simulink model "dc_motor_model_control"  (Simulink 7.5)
settings: Solver=FixedStepDiscrete  StartTime=0.0  StopTime=60  FixedStep=0.001  RelTol=1e-3
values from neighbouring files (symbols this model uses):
  bits = 32    [hexcalc.m]
undefined symbols (not defined in the file or in its folder): bin2dec, Buffer, characters, contain, DiscIntNeverNeededParam, full, is, PWM, Receive, When
libraries: dsPICdrivers x9, simulink x2

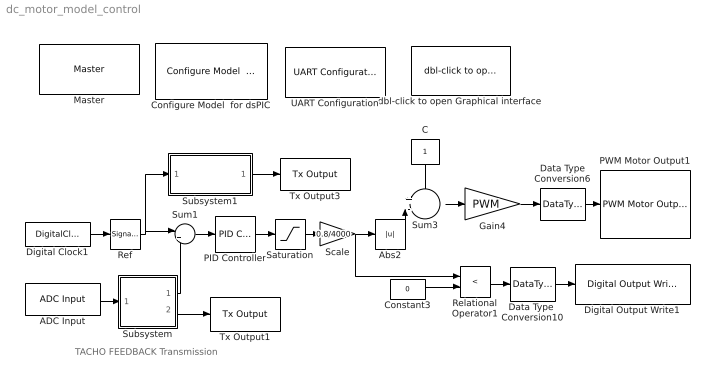
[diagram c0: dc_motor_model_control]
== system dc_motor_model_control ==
  note: TACHO FEEDBACK Transmission
  ADC Input : dsPICdrivers/Peripheral I//O/ADC Input  Tag=dsPIC_ADC  Priority=5  ADC_TYPE=10 bits  ADC_MODE=Continuous sampling & get last channel value  NbrSampleStep=1  VoltRefpopup="AVdd  -  AVss"  OutFormatBitspopup=0000 00dd dddd dddd : Integer  InterruptPriority=6  ANCHANNELS=[3]  MaxName=ANmax = 1023  Rin=1e2  ADCS=1  SAMC=1  Temperature=25  DMAChannel=0  SampleTime=0.001  Status="OK  |  Tsmp=1.600e-007 |  T/Channel=2.080e-006 |  Tall=2.080e-006"  SSRC=auto convert
  Abs2 : Abs  OutDataType=fixdt(1, 16)  OutScaling=2^0
  C : Constant  OutDataType=fixdt(1, 16)  OutScaling=2^0
  Configure Model  for dsPIC : dsPICdrivers/Simulink Configuration/Configure Model  for dsPIC
  Constant3 : Constant  Value=0  OutDataType=fixdt(1, 16)  OutScaling=2^0
  Data Type  Conversion10 : DataTypeConversion  OutDataTypeMode=boolean  OutDataType=fixdt(1, 16)  OutScaling=2^0  OutDataTypeStr=boolean
  Data Type Conversion6 : DataTypeConversion  OutDataTypeMode=uint16  OutDataType=fixdt(1, 16)  OutScaling=2^0  OutDataTypeStr=uint16  SampleTime=0.001
  Digital Clock1 : DigitalClock  SampleTime=0.001
  Digital Output Write1 : dsPICdrivers/Digital I//O/Digital Output Write  Tag=dsPIC_Digital_Output  Priority=5  PORT=D  Pin=[1]  Simultaneous=off  OrderingInOutPopup=None
  Gain4 : Gain  Gain=PWM  ParameterDataType=fixdt(1, 16)  ParameterScaling=2^0  OutDataType=fixdt(1, 16)  OutScaling=2^0  SampleTime=0.001
  Master : dsPICdrivers/Master  Tag=dsPIC_MASTER  Priority=1  TimeStepType=Timer1  picType=30f4012  fcy=6.25e6  Quartz_33f=5e6  PLLActive_33f=off  fcyDesired_33f=0  tmr1="[1  6249  0]"  tmr1Info="Time Step : 0.001  ;   Error : 0%  PR1=6249"  tmr2345="[0  0  0  0]"  tmr2345cfg=[-1 -1 -1 -1]  IOautoConf=on  typePort="[ 0   0   0   0   0   0   0   0   0   0   0   0   0   0   0   0   0   0   0   8   0   0   0   0   0   0   0   0   0   0   0   0   0   0   0   0   0   0   0   0   0   0   0   0   0   0   0   0   0  10   0   0   0   0   0   0   0   0   0   0   0   0   0   0   0   0   0   0   0   0   0   0   0   0   0   0   0   0   0   0   0   0   4   5   0   0   0   0   0   0   0   0   0   0   0   0   0   0   0   0 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"  TRIS="[ 65535  65535  65535  65533  65535  65535  65535 ]"  ADPCFG=0  MasterBusyPort=None  MasterOverloadPort=None  FOSC=HS  ClockSwitchMonitor=Both disabled  TempProtection_33f=TEMP_ON  FPBOR=PBOR_OFF  PWRT=PWRT_OFF  MCLR=MCLR_DIS  ICD=ICS_NONE  JTAGEN=JTAGEN_OFF  PowerSave=off  OverrideFcy=off  NewFcy=1e6  PR2345="[65535  65535  65535  65535]"
  PID Controller : simulink/Continuous/PID Controller  DialogController=pidpack.PIDConfig.pidDDGCreate  DialogControllerArgs=DataTag0  SystemSampleTime=-1  Controller=PID  TimeDomain=Discrete-time  SampleTime=0.001  IntegratorMethod=Forward Euler  FilterMethod=Forward Euler  Form=Parallel  P=2.70860587935341  I=38.2988282363773  D=0.0377965070622529  N=150.289906097433  InitialConditionSource=internal  InitialConditionForIntegrator=0  InitialConditionForFilter=0  ExternalReset=none  LimitOutput=off  UpperSaturationLimit=inf  LowerSaturationLimit=-inf  LinearizeAsGain=off  AntiWindupMode=none  Kb=1  TrackingMode=off  Kt=1  PParamMin=[]  PParamMax=[]  IParamMin=[]  IParamMax=[]  DParamMin=[]  DParamMax=[]  NParamMin=[]  NParamMax=[]  KbParamMin=[]  KbParamMax=[]  KtParamMin=[]  KtParamMax=[]  POutMin=[]  POutMax=[]  IOutMin=[]  IOutMax=[]  DOutMin=[]  DOutMax=[]  NOutMin=[]  NOutMax=[]  KbOutMin=[]  KbOutMax=[]  KtOutMin=[]  KtOutMax=[]  IntegratorOutMin=[]  IntegratorOutMax=[]  FilterOutMin=[]  FilterOutMax=[]  SumOutMin=[]  SumOutMax=[]  SumI1OutMin=[]  SumI1OutMax=[]  SumI2OutMin=[]  SumI2OutMax=[]  SumI3OutMin=[]  SumI3OutMax=[]  SumDOutMin=[]  SumDOutMax=[]  SaturationOutMin=[]  SaturationOutMax=[]  IntegratorContinuousStateAttributes=''  IntegratorStateMustResolveToSignalObject=off  IntegratorRTWStateStorageClass=Auto  FilterContinuousStateAttributes=''  FilterStateMustResolveToSignalObject=off  FilterRTWStateStorageClass=Auto
  PWM Motor Output1 : dsPICdrivers/Peripheral I//O/PWM Motor Output  Tag=dsPIC_PWM_Motor  Priority=5  PWMref=1  PWM12=1  InputEnableChk=off  InputPeriodeChk=off  Channel=[1]  TPeriode=10e-3  PrescalerValue=4  PeriodeInteger=15625  MaxName='PWM'  Centered=off  HChannelON=off  Info="Nbr Bits : 14.9316  ||  PWM = 31250  ||  Prescaler = 4"  Delay=0  IntPriority=5  nbrPwmChannelPIC=3  Status=OK  DeadTimePrescaleA=0  DeadTimePrescaleB=0  DeadTimeInfo=Dead Time A = 0  DTPWM1a=Prescaler A  DTPWM1i=Prescaler A  DTPWM2a=Prescaler A  DTPWM2i=Prescaler A  DTPWM3a=Prescaler A  DTPWM3i=Prescaler A  DTPWM4a=Prescaler A  DTPWM4i=Prescaler A  DTCON1=0  DTCON2=0
  Ref : SignalGenerator  WaveForm=square  TimeSource=Use external signal  Amplitude=2700  Frequency=1/10
  Relational Operator1 : RelationalOperator  Operator=<  LogicOutDataTypeMode=boolean  LogicDataType=fixdt(0, 8)  OutDataTypeStr=boolean
  Saturation : Saturate  UpperLimit=4000  LowerLimit=-4000  OutDataType=fixdt(1, 16)  OutScaling=2^0
  Scale : Gain  Gain=0.8/4000  ParameterDataType=fixdt(1, 16)  ParameterScaling=2^0  OutDataType=fixdt(1, 16)  OutScaling=2^0
  Subsystem : Subsystem
  Subsystem1 : Subsystem
  Sum1 : Sum  Inputs=|+-  OutDataType=fixdt(1, 16)  OutScaling=2^0
  Sum3 : Sum  Inputs=+-  OutDataType=fixdt(1, 16)  OutScaling=2^0
  Tx Output1 : dsPICdrivers/Serial PORT/Tx Output  Tag=dsPIC_TX  Priority=5  UART=1  OrderingInOutPopup=None
  Tx Output3 : dsPICdrivers/Serial PORT/Tx Output  Tag=dsPIC_TX  Priority=5  UART=1  OrderingInOutPopup=None
  UART Configuration : dsPICdrivers/Serial PORT/UART Configuration  Tag=dsPIC_config_UART  Priority=2  UART=1  proposed_BAUD=57600  ALT_TX_RX=off  InterruptTxWhen=When Transmit Buffer is empty  TXInterruptPri=1  TxBufferSize=32  TXEN=on  InterruptRxWhen=When Receive Buffer is full (contain 4 characters)  RXInterruptPri=2  RxBufferSize=32  BAUD=57600  UxBRG=6  Info="UxBRG = 6   ||  Real Baud : 55804   ||  % error : -3.1188  ||  max 5.5804 Bytes / Step"  RealBaud=0
  dbl-click to open Graphical interface : dsPICdrivers/Serial PORT/dbl-click to open Graphical interface  Nothing=0
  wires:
  ADC Input/1 -> Subsystem/1(In1)
  Digital Clock1/1 -> Ref/1
  Ref/1 -> Sum1/1, Subsystem1/1(Ref_in)
  Saturation/1 -> Scale/1
  Scale/1 -> Abs2/1, Relational Operator1/1
  Data Type  Conversion10/1 -> Digital Output Write1/1
  Constant3/1 -> Relational Operator1/2
  Relational Operator1/1 -> Data Type  Conversion10/1
  Data Type Conversion6/1 -> PWM Motor Output1/1
  Gain4/1 -> Data Type Conversion6/1
  C/1 -> Sum3/1
  Sum3/1 -> Gain4/1
  Subsystem/1(FB) -> Sum1/2
  Subsystem/2(Tx) -> Tx Output1/1
  Sum1/1 -> PID Controller/1
  PID Controller/1 -> Saturation/1
  Abs2/1 -> Sum3/2
  Subsystem1/1(Tx) -> Tx Output3/1

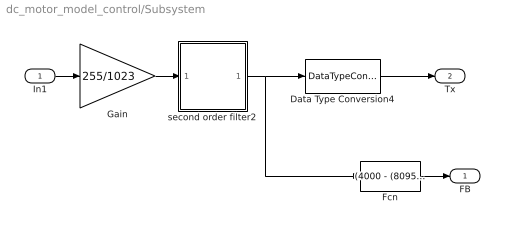
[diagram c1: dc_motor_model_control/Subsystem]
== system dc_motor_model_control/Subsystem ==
  In1 : Inport
  Data Type Conversion4 : DataTypeConversion  OutDataTypeMode=uint8  OutDataType=fixdt(1, 16)  OutScaling=2^0  OutDataTypeStr=uint8  RndMeth=Convergent
  Fcn : Fcn  Expr=(4000 - (8095/204)*u)
  Gain : Gain  Gain=255/1023  ParameterDataType=fixdt(1, 16)  ParameterScaling=2^0  OutDataTypeMode=double  OutDataType=fixdt(1, 16)  OutScaling=2^0  OutDataTypeStr=double
  second order filter2 : Subsystem
  FB : Outport  OutDataType=fixdt(1, 16)  OutScaling=2^0
  Tx : Outport  Port=2  OutDataType=fixdt(1, 16)  OutScaling=2^0
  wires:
  Data Type Conversion4/1 -> Tx/1
  Fcn/1 -> FB/1
  In1/1 -> Gain/1
  second order filter2/1(Out1) -> Fcn/1, Data Type Conversion4/1
  Gain/1 -> second order filter2/1(In1)

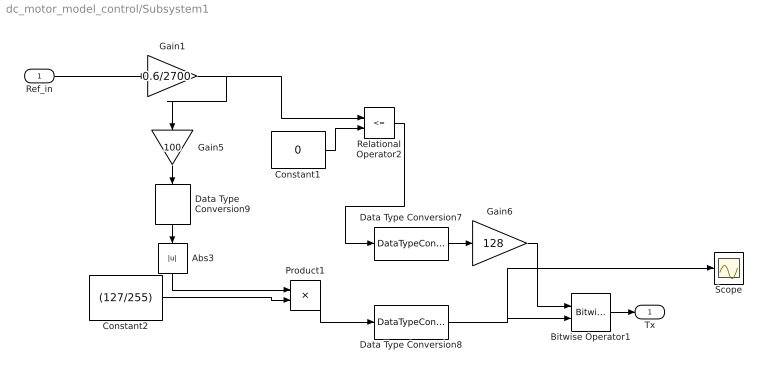
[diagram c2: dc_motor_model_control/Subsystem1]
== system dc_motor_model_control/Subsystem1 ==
  Ref_in : Inport  OutDataType=fixdt(1, 16)  OutScaling=2^0
  Abs3 : Abs  OutDataType=fixdt(1, 16)  OutScaling=2^0
  Bitwise Operator1 : simulink/Logic and Bit Operations/Bitwise Operator  logicop=OR  UseBitMask=off  NumInputPorts=2  BitMask=bin2dec('11011001')  BitMaskRealWorld=Stored Integer
  Constant1 : Constant  Value=0  OutDataType=fixdt(1, 16)  OutScaling=2^0
  Constant2 : Constant  Value=(127/255)  OutDataTypeMode=Specify via dialog  OutDataType=fixdt(1,16)  ConRadixGroup=Best Precision: Vector-wise  OutDataTypeStr=fixdt(1,16)
  Data Type Conversion7 : DataTypeConversion  OutDataTypeMode=uint8  OutDataType=fixdt(1, 16)  OutScaling=2^0  OutDataTypeStr=uint8
  Data Type Conversion8 : DataTypeConversion  OutDataTypeMode=uint8  OutDataType=fixdt(1, 16)  OutScaling=2^0  OutDataTypeStr=uint8
  Data Type Conversion9 : DataTypeConversion  OutDataTypeMode=int8  OutDataType=fixdt(1, 16)  OutScaling=2^0  OutDataTypeStr=int8
  Gain1 : Gain  Gain=0.6/2700  ParameterDataType=fixdt(1, 16)  ParameterScaling=2^0  OutDataType=fixdt(1, 16)  OutScaling=2^0
  Gain5 : Gain  Gain=100  ParameterDataType=fixdt(1, 16)  ParameterScaling=2^0  OutDataTypeMode=int8  OutDataType=fixdt(1, 16)  OutScaling=2^0  OutDataTypeStr=int8
  Gain6 : Gain  Gain=128  ParameterDataType=fixdt(1, 16)  ParameterScaling=2^0  OutDataTypeMode=uint8  OutDataType=fixdt(1, 16)  OutScaling=2^0  OutDataTypeStr=uint8
  Product1 : Product
  Relational Operator2 : RelationalOperator  Operator=<=  LogicOutDataTypeMode=boolean  LogicDataType=fixdt(0, 8)  OutDataTypeStr=boolean
  Scope : Scope
  Tx : Outport
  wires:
  Product1/1 -> Data Type Conversion8/1
  Constant2/1 -> Product1/2
  Data Type Conversion8/1 -> Bitwise Operator1/2, Scope/1
  Data Type Conversion9/1 -> Abs3/1
  Gain5/1 -> Data Type Conversion9/1
  Abs3/1 -> Product1/1
  Constant1/1 -> Relational Operator2/2
  Data Type Conversion7/1 -> Gain6/1
  Gain6/1 -> Bitwise Operator1/1
  Relational Operator2/1 -> Data Type Conversion7/1
  Ref_in/1 -> Gain1/1
  Gain1/1 -> Relational Operator2/1, Gain5/1
  Bitwise Operator1/1 -> Tx/1

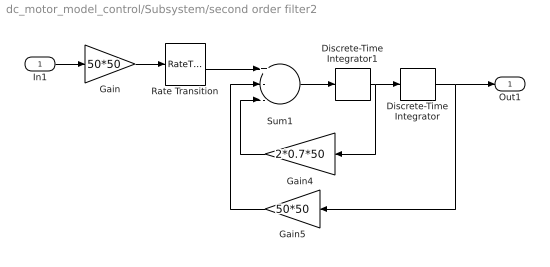
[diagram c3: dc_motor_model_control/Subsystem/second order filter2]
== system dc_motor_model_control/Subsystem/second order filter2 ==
  In1 : Inport  OutDataType=fixdt(1, 16)  OutScaling=2^0
  Discrete-Time Integrator : DiscreteIntegrator  SampleTime=0.001  OutDataTypeMode=double  OutDataType=fixdt(1, 16)  OutScaling=2^0  OutDataTypeStr=double  ICPrevOutput=DiscIntNeverNeededParam  ICPrevScaledInput=DiscIntNeverNeededParam
  Discrete-Time Integrator1 : DiscreteIntegrator  SampleTime=0.001  OutDataTypeMode=double  OutDataType=fixdt(1, 16)  OutScaling=2^0  OutDataTypeStr=double  ICPrevOutput=DiscIntNeverNeededParam  ICPrevScaledInput=DiscIntNeverNeededParam
  Gain : Gain  Gain=50*50  ParameterDataType=fixdt(1, 16)  ParameterScaling=2^0  OutDataTypeMode=double  OutDataType=fixdt(1, 16)  OutScaling=2^0  OutDataTypeStr=double
  Gain4 : Gain  Gain=2*0.7*50  ParameterDataType=fixdt(1, 16)  ParameterScaling=2^0  OutDataTypeMode=double  OutDataType=fixdt(1, 16)  OutScaling=2^0  OutDataTypeStr=double
  Gain5 : Gain  Gain=50*50  ParameterDataType=fixdt(1, 16)  ParameterScaling=2^0  OutDataTypeMode=double  OutDataType=fixdt(1, 16)  OutScaling=2^0  OutDataTypeStr=double
  Rate Transition : RateTransition  Integrity=off  Deterministic=off  OutPortSampleTime=0.001
  Sum1 : Sum  Inputs=+--  OutDataTypeMode=double  OutDataType=fixdt(1, 16)  OutScaling=2^0  OutDataTypeStr=double  SampleTime=0.001
  Out1 : Outport  OutDataType=fixdt(1, 16)  OutScaling=2^0
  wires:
  Rate Transition/1 -> Sum1/1
  In1/1 -> Gain/1
  Gain5/1 -> Sum1/2
  Discrete-Time Integrator/1 -> Out1/1, Gain5/1
  Gain4/1 -> Sum1/3
  Sum1/1 -> Discrete-Time Integrator1/1
  Discrete-Time Integrator1/1 -> Discrete-Time Integrator/1, Gain4/1
  Gain/1 -> Rate Transition/1
